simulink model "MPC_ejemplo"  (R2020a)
settings: Solver=VariableStepAuto  StartTime=0.0  StopTime=10.0  RelTol=1e-3
undefined symbols (not defined in the file): A_T, B_T, C_T, D_T, K_T
libraries: simulink_extras x1, mpclib x1

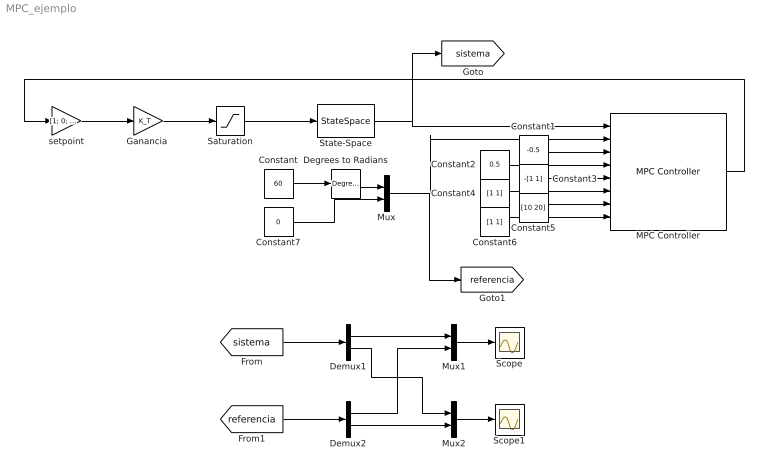
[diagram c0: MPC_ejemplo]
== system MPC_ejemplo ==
  Constant : Constant  Value=60
  Constant1 : Constant  Value=-0.5
  Constant2 : Constant  Value=0.5
  Constant3 : Constant  Value=-[1 1]
  Constant4 : Constant  Value=[1 1]
  Constant5 : Constant  Value=[10 20]
  Constant6 : Constant  Value=[1 1]
  Constant7 : Constant  Value=0
  Degrees to Radians : simulink_extras/Transformations/Degrees to Radians
  Demux1 : Demux  Outputs=2
  Demux2 : Demux  Outputs=2
  "Ganancia " : Gain  Gain=K_T  Multiplication=Matrix(K*u)
  MPC Controller : mpclib/MPC Controller  SCDEnableBlockLinearizationSpecification=on  mpcobj=mpc1  is_multiple=0  enable_value=0  return_u0=off  updateMPCinCallerWorkspace=on  md_inport=off  mv_inport=off  uref_inport=off  return_cost=off  return_mvseq=off  return_qpstatus=off  return_xseq=off  return_state=off  return_ovseq=off  state_inport=off  umin_inport=on  umax_inport=on  ymin_inport=on  ymax_inport=on  cc_inport=off  ywt_inport=on  uwt_inport=on  duwt_inport=off  rhoeps_inport=off  pm_inport=off  MaximumP=10  HorizonChoice=FixedHorizon  n_ts=0.1  n_p=10  n_mv=1  n_md=0  n_ud=0  n_mo=2  n_uo=0  BlockDataType=double  SampleTimeInherited=off  switch_inport=off
  Mux : Mux  Inputs=2
  Mux1 : Mux  Inputs=2
  Mux2 : Mux  Inputs=2
  Saturation : Saturate  UpperLimit=7  LowerLimit=-7
  Scope : Scope
  Scope1 : Scope
  State-Space : StateSpace  A=A_T  B=B_T  C=C_T  D=D_T  InitialCondition=[0;0;0;0]
  setpoint : Gain  Gain=[1; 0; 0; 0]
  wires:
  State-Space/1 -> [sistema], MPC Controller/1
  Constant/1 -> Degrees to Radians/1
  setpoint/1 -> "Ganancia "/1
  Saturation/1 -> State-Space/1
  "Ganancia "/1 -> Saturation/1
  MPC Controller/1 -> setpoint/1
  Constant1/1 -> MPC Controller/3
  Constant2/1 -> MPC Controller/4
  Constant3/1 -> MPC Controller/5
  Constant4/1 -> MPC Controller/6
  Constant5/1 -> MPC Controller/7
  Constant6/1 -> MPC Controller/8
  Degrees to Radians/1 -> Mux/1
  Mux/1 -> [referencia], MPC Controller/2
  Constant7/1 -> Mux/2
  [sistema] -> Demux1/1
  [referencia] -> Demux2/1
  Demux1/1 -> Mux1/1
  Demux2/1 -> Mux1/2
  Demux1/2 -> Mux2/1
  Demux2/2 -> Mux2/2
  Mux2/1 -> Scope1/1
  Mux1/1 -> Scope/1
